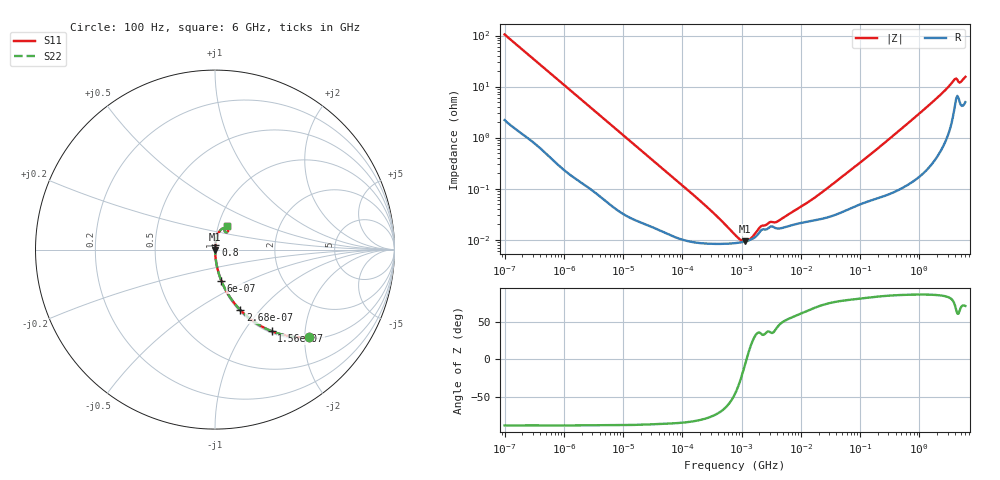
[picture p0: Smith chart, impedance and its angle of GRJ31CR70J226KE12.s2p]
!Murata Part Number: GRJ31CR70J226KE12
!These Parameters are Measured in Series Mode Connection
!Data Generated on Jun 19, 2026
!  o--ll--o
!Port1  Port2
!  o------o
!Operation Temp=25[degC], DC Bias Voltage=0[V]
!Freq. Start=100[Hz] Stop=6[GHz] 401[Steps]
# Hz S RI R 50
!Freq.(Hz) S11(Real) S11(Imag) S21(Real) S21(Imag) S12(Real) S12(Imag) S22(Real) S22(Imag)
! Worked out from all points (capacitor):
!   401 points, 100 Hz to 6 GHz, reference 50 ohm
!   read as one part in series: C = 15.1 uF near 109 Hz
!   lowest |Z| = 9.26 mohm at 1.159 MHz (marker M1)
!   series resonance near 1.213 MHz, so ESL is about 1.1 nH
!   S11 on the Smith chart (normalised r, x): 100 Hz: 1.04, -2.10; 156 Hz: 1.03, -1.35; 268 Hz: 1.02, -0.79; 600 Hz: 1.01, -0.36; 800 MHz: 1.00, +0.05; 6 GHz: 1.10, +0.29
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100  0.5238 -0.4891  0.4762 0.4891  0.4762 0.4891  0.5238 -0.4891
156  0.3162 -0.4544  0.6838 0.4544  0.6838 0.4544  0.3162 -0.4544
268  0.1417 -0.3376  0.8583 0.3376  0.8583 0.3376  0.1417 -0.3376
383  0.0773 -0.2558  0.9227 0.2558  0.9227 0.2558  0.0773 -0.2558
600  0.0348 -0.1726  0.9652 0.1726  0.9652 0.1726  0.0348 -0.1726
2008  0.00422 -0.0541  0.9958 0.0541  0.9958 0.0541  0.00422 -0.0541
40335  0.000162 -0.00283  0.9998 0.00283  0.9998 0.00283  0.000162 -0.00283
264476  8.35e-05 -0.000422  0.9999 0.000422  0.9999 0.000422  8.35e-05 -0.000422
774597  8.53e-05 -8.99e-05  0.9999 8.99e-05  0.9999 8.99e-05  8.53e-05 -8.99e-05
926525  8.75e-05 -5.29e-05  0.9999 5.29e-05  0.9999 5.29e-05  8.75e-05 -5.29e-05
1159002  9.22e-05 -8.8e-06  0.9999 8.8e-06  0.9999 8.8e-06  9.22e-05 -8.8e-06
1449809  0.000101 3.56e-05  0.9999 -3.56e-05  0.9999 -3.56e-05  0.000101 3.56e-05
2169299  0.000154 0.000103  0.9998 -0.000103  0.9998 -0.000103  0.000154 0.000103
3103719  0.000181 0.00013  0.9998 -0.00013  0.9998 -0.00013  0.000181 0.00013
4060267  0.000165 0.000157  0.9998 -0.000157  0.9998 -0.000157  0.000165 0.000157
1.555665e7  0.000234 0.000568  0.9998 -0.000568  0.9998 -0.000568  0.000234 0.000568
3.124326e8  0.000867 0.00939  0.9991 -0.00939  0.9991 -0.00939  0.000867 0.00939
8.000355e8  0.00195 0.0236  0.998 -0.0236  0.998 -0.0236  0.00195 0.0236
2.562649e9  0.0129 0.0769  0.9871 -0.0769  0.9871 -0.0769  0.0129 0.0769
3.8344e9  0.0459 0.1193  0.9541 -0.1193  0.9541 -0.1193  0.0459 0.1193
5.016141e9  0.0535 0.1042  0.9465 -0.1042  0.9465 -0.1042  0.0535 0.1042
6e9  0.0655 0.1311  0.9345 -0.1311  0.9345 -0.1311  0.0655 0.1311
